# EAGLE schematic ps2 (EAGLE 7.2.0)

## Sheet 1 of 3: KL25Z Connections
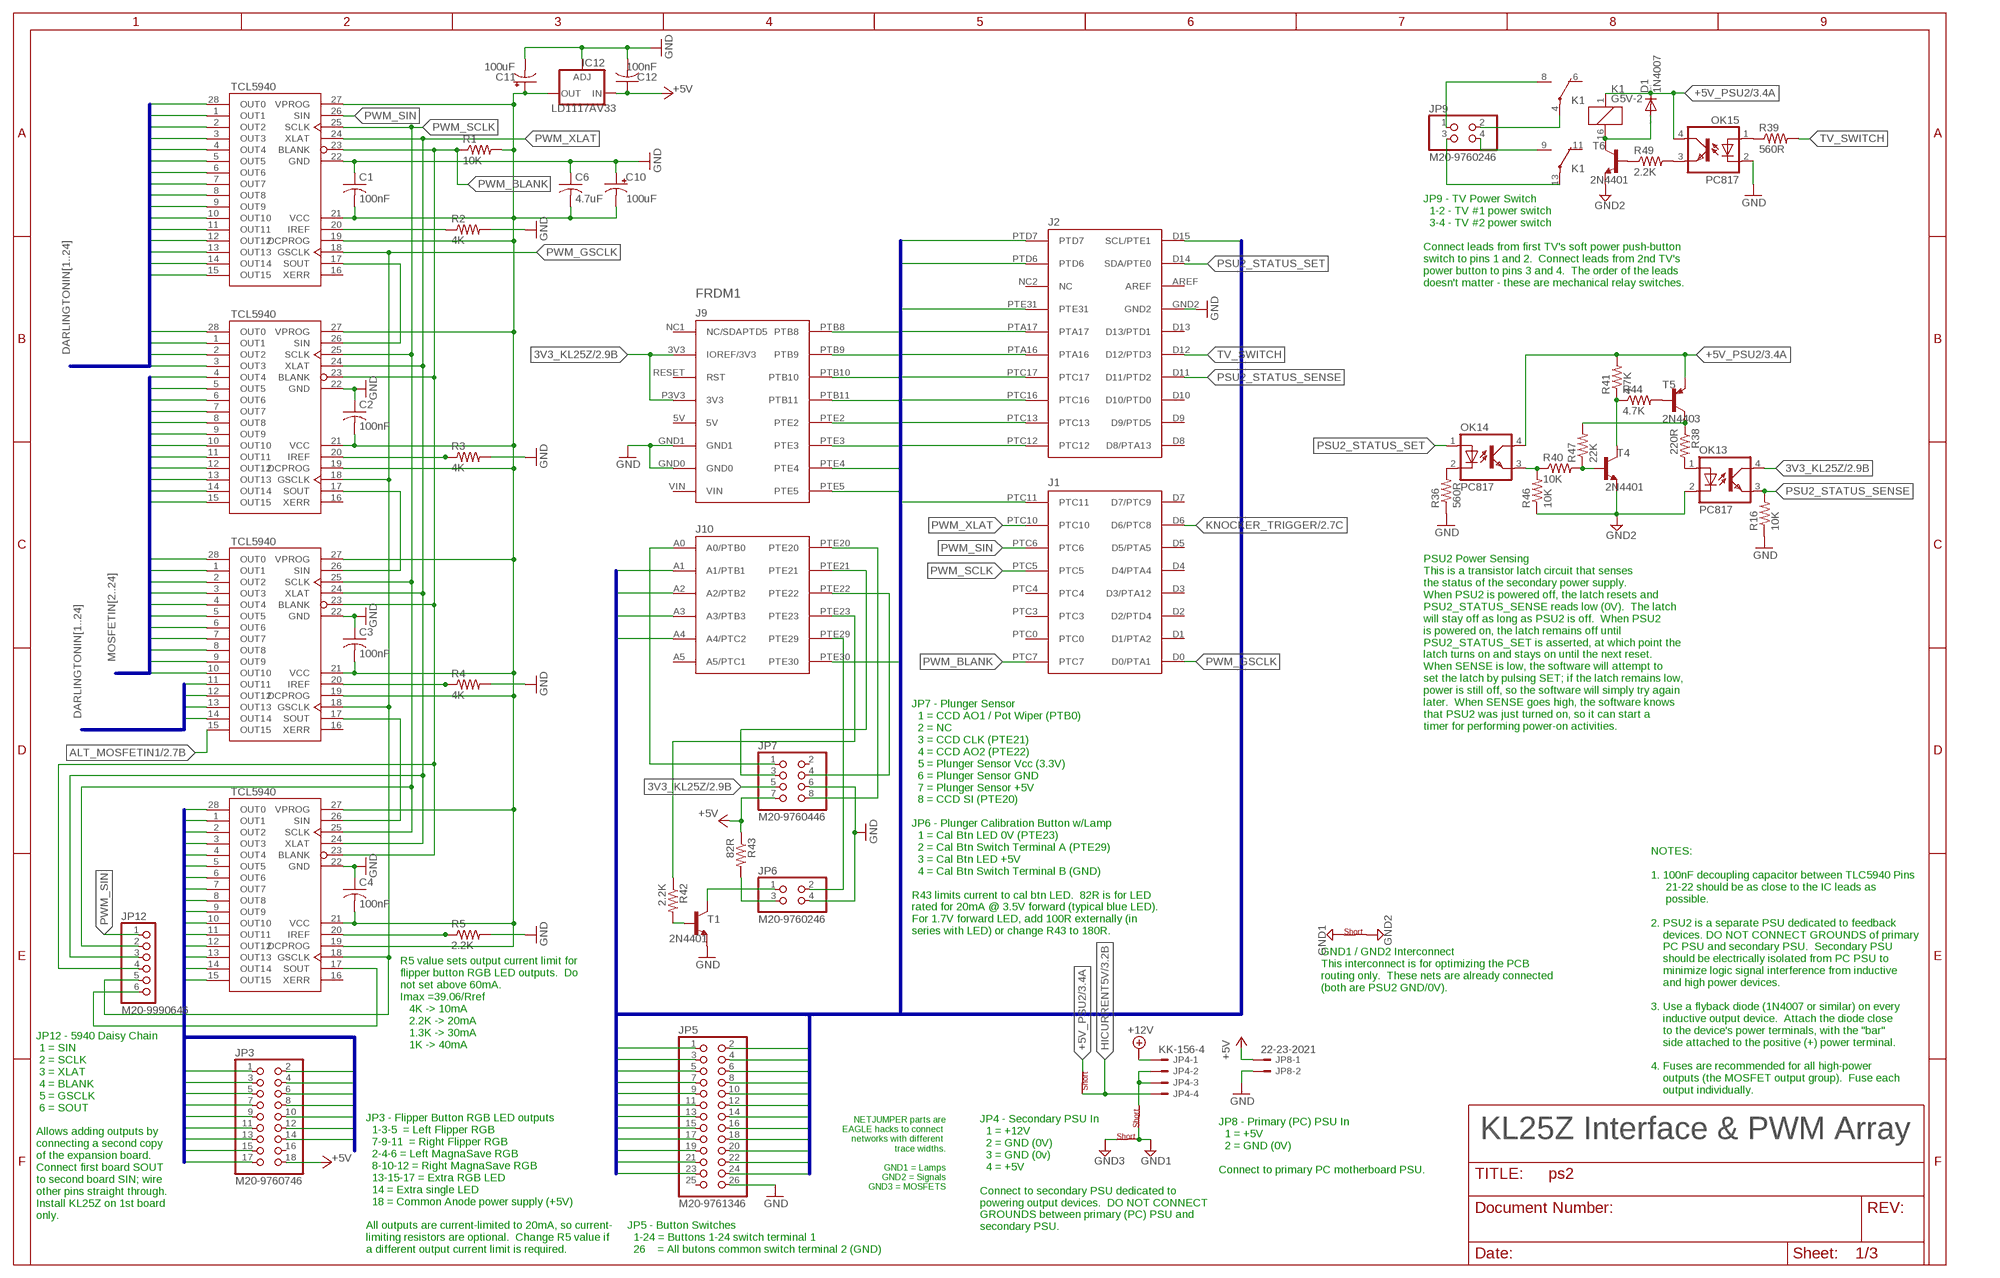
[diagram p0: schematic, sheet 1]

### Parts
C1  100nF  C-US025-024X044  [C025-024X044]
C2  100nF  C-US025-024X044  [C025-024X044]
C3  100nF  C-US025-024X044  [C025-024X044]
C4  100nF  C-US025-024X044  [C025-024X044]
C6  4.7uF  C-US025-024X044  [C025-024X044]
C10  100uF  CPOL-USE2.5-5  [E2,5-5]
C11  100uF  CPOL-USE2.5-5  [E2,5-5]
C12  100nF  C-US025-024X044  [C025-024X044]
D1  1N4007  DIODE-DO41-10  [DO41-10]
FRDM1  KL25Z  FRDM-KL25ZNORMAL  [FRDM_KL25Z_NORMAL]
IC1  TLC5940NT  TCL5940TLC5940NT  [DIP28]
IC2  TLC5940NT  TCL5940TLC5940NT  [DIP28]
IC3  TLC5940NT  TCL5940TLC5940NT  [DIP28]
IC4  TLC5940NT  TCL5940TLC5940NT  [DIP28]
IC12  LD1117AV33  LD117A  [TO220S]
JP3  M20-9760746  PINHD-2X9  [2X09]
JP4  KK-156-4  [KK-156-4]
JP5  M20-9761346  PINHD-2X13  [2X13]
JP6  M20-9760246  PINHD-2X2  [2X02]
JP7  M20-9760446  PINHD-2X4  [2X04]
JP8  22-23-2021  [22-23-2021]
JP9  M20-9760246  PINHD-2X2  [2X02]
JP12  M20-9990646  PINHD-1X6  [1X06]
K1  G5V-2  [G5V-2]
OK13  PC817  [DIL04]
OK14  PC817  [DIL04]
OK15  PC817  [DIL04]
R1  10K  R-US_0207/10  [0207/10]
R2  4K  R-US_0207/10  [0207/10]
R3  4K  R-US_0207/10  [0207/10]
R4  4K  R-US_0207/10  [0207/10]
R5  2.2K  R-US_0207/10  [0207/10]
R16  10K  R-US_0207/10  [0207/10]
R36  560R  R-US_0207/10  [0207/10]
R38  220R  R-US_0207/10  [0207/10]
R39  560R  R-US_0207/10  [0207/10]
R40  10K  R-US_0207/10  [0207/10]
R41  4.7K  R-US_0207/10  [0207/10]
R42  2.2K  R-US_0207/10  [0207/10]
R43  82R  R-US_0207/10  [0207/10]
R44  4.7K  R-US_0207/10  [0207/10]
R46  10K  R-US_0207/10  [0207/10]
R47  22K  R-US_0207/10  [0207/10]
R49  2.2K  R-US_0207/10  [0207/10]
T1  2N4401  2N4401-NPN-TO92-EBC  [TO92-EBC]
T4  2N4401  2N4401-NPN-TO92-EBC  [TO92-EBC]
T5  2N4403  2N4403-PNP-TO92-EBC  [TO92-EBC]
T6  2N4401  2N4401-NPN-TO92-EBC  [TO92-EBC]
U$1  NETJUMPER  [JP0]
U$2  NETJUMPER  [JP0]
U$3  NETJUMPER  [JP0]
U$4  NETJUMPER  [JP0]

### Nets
3V3_KL25Z: FRDM1.3V3(IOREF/3V3) FRDM1.P3V3(3V3) JP7.5 OK13.4(COL) ; also sheet 2
+5V [+5V]: C12.1 IC12.3(IN) JP3.18 JP7.7 JP8.1 R43.1 ; also sheet 2,3
+5V_PSU2: D1.C K1.1 OK14.4(COL) OK15.4(COL) R41.2 T5.E U$1.P$2 ; also sheet 3
+12V: JP4.1 ; also sheet 2
ALT_MOSFETIN1: IC3.15(OUT15) ; also sheet 2
DARLINGTONIN1: IC1.28(OUT0) ; also sheet 3
DARLINGTONIN2: IC1.1(OUT1) ; also sheet 3
DARLINGTONIN3: IC1.2(OUT2) ; also sheet 3
DARLINGTONIN4: IC1.3(OUT3) ; also sheet 3
DARLINGTONIN5: IC1.4(OUT4) ; also sheet 3
DARLINGTONIN6: IC1.5(OUT5) ; also sheet 3
DARLINGTONIN7: IC1.6(OUT6) ; also sheet 3
DARLINGTONIN8: IC1.7(OUT7) ; also sheet 3
DARLINGTONIN9: IC1.8(OUT8) ; also sheet 3
DARLINGTONIN10: IC1.9(OUT9) ; also sheet 3
DARLINGTONIN11: IC1.10(OUT10) ; also sheet 3
DARLINGTONIN12: IC1.11(OUT11) ; also sheet 3
DARLINGTONIN13: IC1.12(OUT12) ; also sheet 3
DARLINGTONIN14: IC1.13(OUT13) ; also sheet 3
DARLINGTONIN15: IC1.14(OUT14) ; also sheet 3
DARLINGTONIN16: IC1.15(OUT15) ; also sheet 3
DARLINGTONIN17: IC2.28(OUT0) ; also sheet 3
DARLINGTONIN18: IC2.1(OUT1) ; also sheet 3
DARLINGTONIN19: IC2.2(OUT2) ; also sheet 3
DARLINGTONIN20: IC2.3(OUT3) ; also sheet 3
DARLINGTONIN21: IC3.11(OUT11) ; also sheet 3
DARLINGTONIN22: IC3.12(OUT12) ; also sheet 3
DARLINGTONIN23: IC3.13(OUT13) ; also sheet 3
DARLINGTONIN24: IC3.14(OUT14) ; also sheet 3
FLIPPER_RGB1: IC4.28(OUT0) JP3.1
FLIPPER_RGB2: IC4.1(OUT1) JP3.3
FLIPPER_RGB3: IC4.2(OUT2) JP3.5
FLIPPER_RGB4: IC4.3(OUT3) JP3.7
FLIPPER_RGB5: IC4.4(OUT4) JP3.9
FLIPPER_RGB6: IC4.5(OUT5) JP3.11
FLIPPER_RGB7: IC4.6(OUT6) JP3.2
FLIPPER_RGB8: IC4.7(OUT7) JP3.4
FLIPPER_RGB9: IC4.8(OUT8) JP3.6
FLIPPER_RGB10: IC4.9(OUT9) JP3.8
FLIPPER_RGB11: IC4.10(OUT10) JP3.10
FLIPPER_RGB12: IC4.11(OUT11) JP3.12
FLIPPER_RGB13: IC4.12(OUT12) JP3.13
FLIPPER_RGB14: IC4.13(OUT13) JP3.15
FLIPPER_RGB15: IC4.14(OUT14) JP3.17
FLIPPER_RGB16: IC4.15(OUT15) JP3.14
GND [GND]: C1.1 C2.1 C3.1 C4.1 C6.1 C10.+ C11.- C12.2 FRDM1.GND0 FRDM1.GND1 FRDM1.GND2 IC1.22(GND) IC2.22(GND) IC3.22(GND) IC4.22(GND) IC12.1(ADJ) JP5.26 JP6.4 JP7.6 JP8.2 OK15.2(C) R2.2 R3.2 R4.2 R5.2 R16.1 R36.1 T1.E ; also sheet 2
GND1 [Lamp Power & Ground]: U$2.P$2 U$3.P$2 U$4.P$1 ; also sheet 3
GND2: OK13.2(C) R46.1 T4.E T6.E U$3.P$1
GND3 [MOSFET Power & Ground]: U$4.P$2 ; also sheet 2
HICURRENT5V [Lamp Power & Ground]: JP4.4 U$1.P$1 ; also sheet 3
KEYS1: FRDM1.A4(A4/PTC2) JP5.1
KEYS2: FRDM1.A3(A3/PTB3) JP5.2
KEYS3: FRDM1.A2(A2/PTB2) JP5.3
KEYS4: FRDM1.A1(A1/PTB1) JP5.4
KEYS5: FRDM1.PTE30 JP5.5
KEYS6: FRDM1.PTC11 JP5.6
KEYS7: FRDM1.PTE5 JP5.7
KEYS8: FRDM1.PTE4 JP5.8
KEYS9: FRDM1.PTE3 JP5.9
KEYS10: FRDM1.PTE2 JP5.10
KEYS11: FRDM1.PTB11 JP5.11
KEYS12: FRDM1.PTB10 JP5.12
KEYS13: FRDM1.PTB9 JP5.13
KEYS14: FRDM1.PTB8 JP5.14
KEYS15: FRDM1.PTC12 JP5.15
KEYS16: FRDM1.PTC13 JP5.16
KEYS17: FRDM1.PTC16 JP5.17
KEYS18: FRDM1.PTC17 JP5.18
KEYS19: FRDM1.PTA16 JP5.19
KEYS20: FRDM1.PTA17 JP5.20
KEYS21: FRDM1.PTE31 JP5.21
KEYS22: FRDM1.PTD6 JP5.22
KEYS23: FRDM1.PTD7 JP5.23
KEYS24: FRDM1.D15(SCL/PTE1) JP5.24
KNOCKER_TRIGGER: FRDM1.D6(D6/PTC8) ; also sheet 2
MOSFETIN2: IC2.4(OUT4) ; also sheet 2
MOSFETIN3: IC2.5(OUT5) ; also sheet 2
MOSFETIN4: IC2.6(OUT6) ; also sheet 2
MOSFETIN5: IC2.7(OUT7) ; also sheet 2
MOSFETIN6: IC2.8(OUT8) ; also sheet 2
MOSFETIN7: IC2.9(OUT9) ; also sheet 2
MOSFETIN8: IC2.10(OUT10) ; also sheet 2
MOSFETIN9: IC2.11(OUT11) ; also sheet 2
MOSFETIN10: IC2.12(OUT12) ; also sheet 2
MOSFETIN11: IC2.13(OUT13) ; also sheet 2
MOSFETIN12: IC2.14(OUT14) ; also sheet 2
MOSFETIN13: IC2.15(OUT15) ; also sheet 2
MOSFETIN14: IC3.28(OUT0) ; also sheet 2
MOSFETIN15: IC3.1(OUT1) ; also sheet 2
MOSFETIN16: IC3.2(OUT2) ; also sheet 2
MOSFETIN17: IC3.3(OUT3) ; also sheet 2
MOSFETIN18: IC3.4(OUT4) ; also sheet 2
MOSFETIN19: IC3.5(OUT5) ; also sheet 2
MOSFETIN20: IC3.6(OUT6) ; also sheet 2
MOSFETIN21: IC3.7(OUT7) ; also sheet 2
MOSFETIN22: IC3.8(OUT8) ; also sheet 2
MOSFETIN23: IC3.9(OUT9) ; also sheet 2
MOSFETIN24: IC3.10(OUT10) ; also sheet 2
N$1: IC1.17(SOUT) IC2.26(SIN)
N$2: IC2.17(SOUT) IC3.26(SIN)
N$3: IC3.17(SOUT) IC4.26(SIN)
N$5: OK15.1(A) R39.1
N$8: R38.1 R47.2 T5.C
N$10: OK13.1(A) R38.2
N$11: OK15.3(EMIT) R49.2
N$12: R49.1 T6.B
N$13: R44.2 T5.B
N$14: R41.1 R44.1 T4.C
N$15: D1.A K1.16 T6.C
N$16: JP9.2 K1.4(1:P)
N$17: IC1.20(IREF) R2.1
N$18: IC2.20(IREF) R3.1
N$19: IC3.20(IREF) R4.1
N$20: IC4.20(IREF) R5.1
N$21: FRDM1.A0(A0/PTB0) JP7.1
N$26: FRDM1.PTE20 JP7.8
N$34: FRDM1.PTE21 JP7.3
N$38: FRDM1.PTE29 JP6.2
N$41: FRDM1.PTE23 R42.1
N$43: OK14.3(EMIT) R40.1 R46.2
N$50: JP9.1 K1.8(1:S)
N$61: OK14.2(C) R36.2
N$68: C1.2 C2.2 C3.2 C4.2 C6.2 C10.- C11.+ IC1.19(DCPROG) IC1.21(VCC) IC1.27(VPROG) IC2.19(DCPROG) IC2.21(VCC) IC2.27(VPROG) IC3.19(DCPROG) IC3.21(VCC) IC3.27(VPROG) IC4.19(DCPROG) IC4.21(VCC) IC4.27(VPROG) IC12.2(OUT) R1.2
N$70: JP4.2 JP4.3 U$2.P$1
N$75: FRDM1.PTE22 JP7.4
N$76: IC4.17(SOUT) JP12.6
N$85: R40.2 R47.1 T4.B
N$86: JP9.4 K1.9(2:S)
N$87: JP9.3 K1.13(2:P)
N$88 [+5V]: JP6.3 R43.2
N$89: JP6.1 T1.C
N$100: R42.2 T1.B
PSU2_STATUS_SENSE: FRDM1.D11(D11/PTD2) OK13.3(EMIT) R16.2
PSU2_STATUS_SET: FRDM1.D14(SDA/PTE0) OK14.1(A)
PWM_BLANK: FRDM1.PTC7 IC1.23(BLANK) IC2.23(BLANK) IC3.23(BLANK) IC4.23(BLANK) JP12.4 R1.1
PWM_GSCLK: FRDM1.D0(D0/PTA1) IC1.18(GSCLK) IC2.18(GSCLK) IC3.18(GSCLK) IC4.18(GSCLK) JP12.5
PWM_SCLK: FRDM1.PTC5 IC1.25(SCLK) IC2.25(SCLK) IC3.25(SCLK) IC4.25(SCLK) JP12.2
PWM_SIN: FRDM1.PTC6 IC1.26(SIN) JP12.1
PWM_XLAT: FRDM1.PTC10 IC1.24(XLAT) IC2.24(XLAT) IC3.24(XLAT) IC4.24(XLAT) JP12.3
TV_SWITCH: FRDM1.D12(D12/PTD3) R39.2
Unconnected: FRDM1.5V FRDM1.A5(A5/PTC1) FRDM1.AREF FRDM1.D1(D1/PTA2) FRDM1.D2(D2/PTD4) FRDM1.D3(D3/PTA12) FRDM1.D4(D4/PTA4) FRDM1.D5(D5/PTA5) FRDM1.D7(D7/PTC9) FRDM1.D8(D8/PTA13) FRDM1.D9(D9/PTD5) FRDM1.D10(D10/PTD0) FRDM1.D13(D13/PTD1) FRDM1.NC1(NC/SDAPTD5) FRDM1.NC2(NC) FRDM1.PTC0 FRDM1.PTC3 FRDM1.PTC4 FRDM1.RESET(RST) FRDM1.VIN IC1.16(XERR) IC2.16(XERR) IC3.16(XERR) IC4.16(XERR) JP3.16 JP5.25 JP7.2 K1.6(1:O) K1.11(2:O)

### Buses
FLIPPER_RGB[1..17]
KEYS[1..24]
MOSFETIN[2..24]
DARLINGTONIN[1..24]

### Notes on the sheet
- JP9 - TV Power Switch
    1-2 - TV #1 power switch
    3-4 - TV #2 power switch
  
  Connect leads from first TV's soft power push-button
  switch to pins 1 and 2.  Connect leads from 2nd TV's
  power button to pins 3 and 4.  The order of the leads
  doesn't matter - these are mechanical relay switches.
- PSU2 Power Sensing
  This is a transistor latch circuit that senses
  the status of the secondary power supply.
  When PSU2 is powered off, the latch resets and
  PSU2_STATUS_SENSE reads low (0V).  The latch
  will stay off as long as PSU2 is off.  When PSU2
  is powered on, the latch remains off until 
  PSU2_STATUS_SET is asserted, at which point the
  latch turns on and stays on until the next reset.
  When SENSE is low, the software will attempt to
  set the latch by pulsing SET; if the latch remains low,
  power is still off, so the software will simply try again
  later.  When SENSE goes high, the software knows
  that PSU2 was just turned on, so it can start a
  timer for performing power-on activities.
- JP7 - Plunger Sensor
    1 = CCD AO1 / Pot Wiper (PTB0)
    2 = NC
    3 = CCD CLK (PTE21)
    4 = CCD AO2 (PTE22)
    5 = Plunger Sensor Vcc (3.3V)
    6 = Plunger Sensor GND
    7 = Plunger Sensor +5V
    8 = CCD SI (PTE20)
  
  JP6 - Plunger Calibration Button w/Lamp
    1 = Cal Btn LED 0V (PTE23)
    2 = Cal Btn Switch Terminal A (PTE29)
    3 = Cal Btn LED +5V
    4 = Cal Btn Switch Terminal B (GND)
  
  R43 limits current to cal btn LED.  82R is for LED
  rated for 20mA @ 3.5V forward (typical blue LED).
  For 1.7V forward LED, add 100R externally (in
  series with LED) or change R43 to 180R.
- GND1 / GND2 Interconnect
  This interconnect is for optimizing the PCB 
  routing only.  These nets are already connected
  (both are PSU2 GND/0V).
- R5 value sets output current limit for 
  flipper button RGB LED outputs.  Do
  not set above 60mA.
  Imax =39.06/Rref
     4K -> 10mA
     2.2K -> 20mA
     1.3K -> 30mA
     1K -> 40mA
- NOTES:
  
  1. 100nF decoupling capacitor between TLC5940 Pins
       21-22 should be as close to the IC leads as 
       possible.
  
  2. PSU2 is a separate PSU dedicated to feedback
      devices. DO NOT CONNECT GROUNDS of primary
      PC PSU and secondary PSU.  Secondary PSU 
      should be electrically isolated from PC PSU to
      minimize logic signal interference from inductive 
      and high power devices.
  
  3. Use a flyback diode (1N4007 or similar) on every
      inductive output device.  Attach the diode close
      to the device's power terminals, with the "bar"
      side attached to the positive (+) power terminal.
  
  4. Fuses are recommended for all high-power
      outputs (the MOSFET output group).  Fuse each
      output individually.
- NETJUMPER parts are
  EAGLE hacks to connect 
  networks with different 
  trace widths.
  
  GND1 = Lamps
  GND2 = Signals
  GND3 = MOSFETS
- KL25Z Interface & PWM Array
- JP8 - Primary (PC) PSU In
    1 = +5V
    2 = GND (0V)
  
  Connect to primary PC motherboard PSU.
- JP12 - 5940 Daisy Chain
   1 = SIN
   2 = SCLK
   3 = XLAT
   4 = BLANK
   5 = GSCLK
   6 = SOUT
  
  Allows adding outputs by
  connecting a second copy
  of the expansion board.
  Connect first board SOUT
  to second board SIN; wire
  other pins straight through.
  Install KL25Z on 1st board
  only.
- JP4 - Secondary PSU In
    1 = +12V
    2 = GND (0V)
    3 = GND (0v)
    4 = +5V
  
  Connect to secondary PSU dedicated to
  powering output devices.  DO NOT CONNECT
  GROUNDS between primary (PC) PSU and
  secondary PSU.
- JP3 - Flipper Button RGB LED outputs
    1-3-5  = Left Flipper RGB
    7-9-11  = Right Flipper RGB
    2-4-6 = Left MagnaSave RGB
    8-10-12 = Right MagnaSave RGB
    13-15-17 = Extra RGB LED
    14 = Extra single LED
    18 = Common Anode power supply (+5V)
  
  All outputs are current-limited to 20mA, so current-
  limiting resistors are optional.  Change R5 value if
  a different output current limit is required.
- JP5 - Button Switches
    1-24 = Buttons 1-24 switch terminal 1
    26    = All butons common switch terminal 2 (GND)

## Sheet 2 of 3: MOSFET Outputs
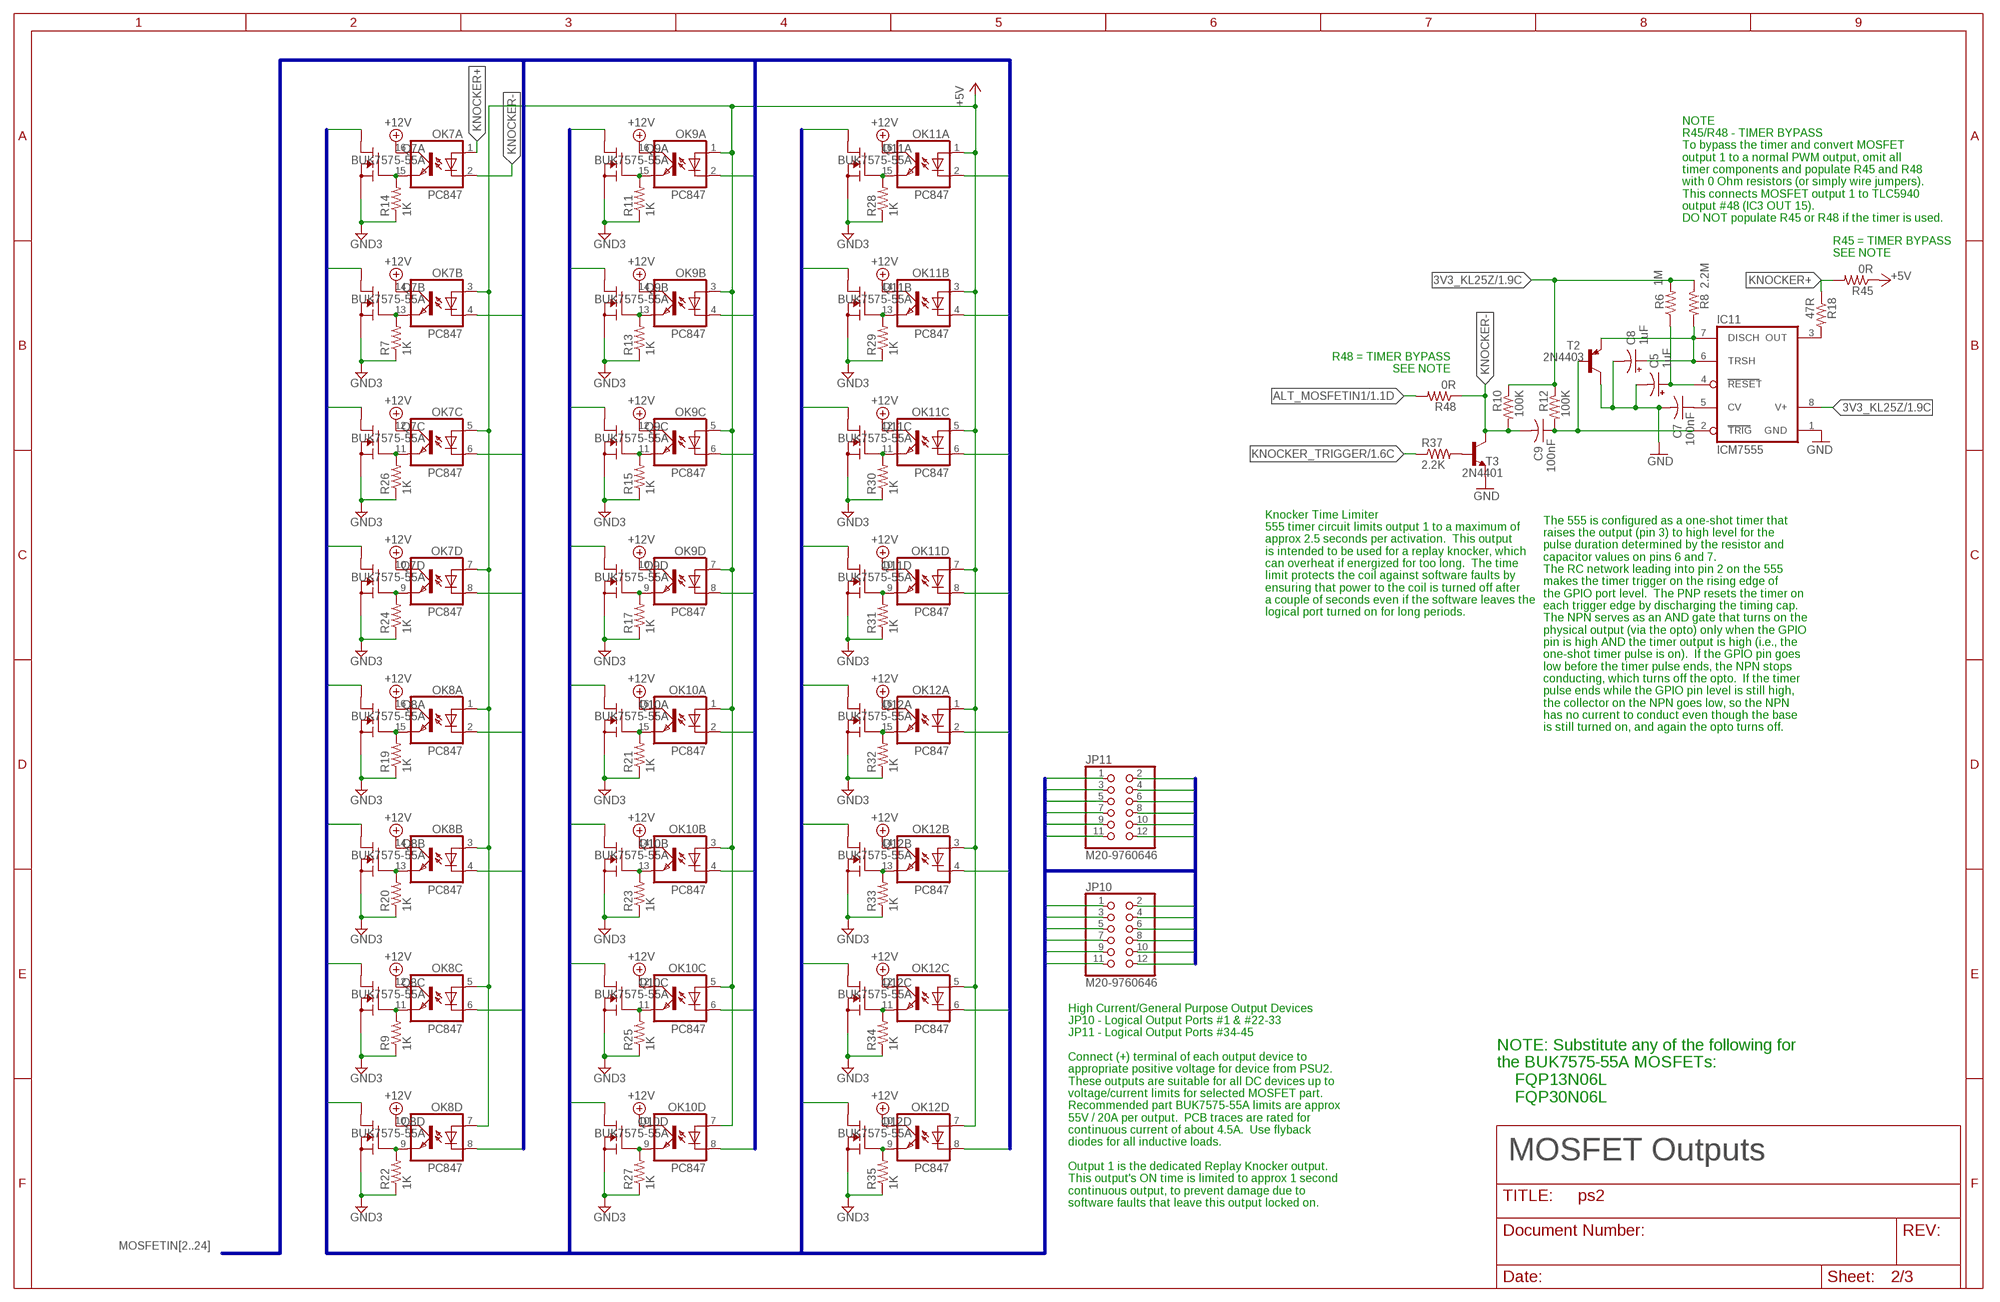
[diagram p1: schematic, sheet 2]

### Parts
C5  1uF  CPOL-USE2.5-5  [E2,5-5]
C7  100nF  C-US025-024X044  [C025-024X044]
C8  1uF  CPOL-USE2.5-5  [E2,5-5]
C9  100nF  C-US025-024X044  [C025-024X044]
IC11  ICM7555  [DIL08]
JP10  M20-9760646  PINHD-2X6  [2X06]
JP11  M20-9760646  PINHD-2X6  [2X06]
OK7  PC847  [DIL16]
OK8  PC847  [DIL16]
OK9  PC847  [DIL16]
OK10  PC847  [DIL16]
OK11  PC847  [DIL16]
OK12  PC847  [DIL16]
Q7A  BUK7575-55A  [TO220BV]
Q7B  BUK7575-55A  [TO220BV]
Q7C  BUK7575-55A  [TO220BV]
Q7D  BUK7575-55A  [TO220BV]
Q8A  BUK7575-55A  [TO220BV]
Q8B  BUK7575-55A  [TO220BV]
Q8C  BUK7575-55A  [TO220BV]
Q8D  BUK7575-55A  [TO220BV]
Q9A  BUK7575-55A  [TO220BV]
Q9B  BUK7575-55A  [TO220BV]
Q9C  BUK7575-55A  [TO220BV]
Q9D  BUK7575-55A  [TO220BV]
Q10A  BUK7575-55A  [TO220BV]
Q10B  BUK7575-55A  [TO220BV]
Q10C  BUK7575-55A  [TO220BV]
Q10D  BUK7575-55A  [TO220BV]
Q11A  BUK7575-55A  [TO220BV]
Q11B  BUK7575-55A  [TO220BV]
Q11C  BUK7575-55A  [TO220BV]
Q11D  BUK7575-55A  [TO220BV]
Q12A  BUK7575-55A  [TO220BV]
Q12B  BUK7575-55A  [TO220BV]
Q12C  BUK7575-55A  [TO220BV]
Q12D  BUK7575-55A  [TO220BV]
R6  1M  R-US_0207/10  [0207/10]
R7  1K  R-US_0207/10  [0207/10]
R8  2.2M  R-US_0207/10  [0207/10]
R9  1K  R-US_0207/10  [0207/10]
R10  100K  R-US_0207/10  [0207/10]
R11  1K  R-US_0207/10  [0207/10]
R12  100K  R-US_0207/10  [0207/10]
R13  1K  R-US_0207/10  [0207/10]
R14  1K  R-US_0207/10  [0207/10]
R15  1K  R-US_0207/10  [0207/10]
R17  1K  R-US_0207/10  [0207/10]
R18  47R  R-US_0207/10  [0207/10]
R19  1K  R-US_0207/10  [0207/10]
R20  1K  R-US_0207/10  [0207/10]
R21  1K  R-US_0207/10  [0207/10]
R22  1K  R-US_0207/10  [0207/10]
R23  1K  R-US_0207/10  [0207/10]
R24  1K  R-US_0207/10  [0207/10]
R25  1K  R-US_0207/10  [0207/10]
R26  1K  R-US_0207/10  [0207/10]
R27  1K  R-US_0207/10  [0207/10]
R28  1K  R-US_0207/10  [0207/10]
R29  1K  R-US_0207/10  [0207/10]
R30  1K  R-US_0207/10  [0207/10]
R31  1K  R-US_0207/10  [0207/10]
R32  1K  R-US_0207/10  [0207/10]
R33  1K  R-US_0207/10  [0207/10]
R34  1K  R-US_0207/10  [0207/10]
R35  1K  R-US_0207/10  [0207/10]
R37  2.2K  R-US_0207/10  [0207/10]
R45  0R  R-US_0204/2V  [0204V]
R48  0R  R-US_0204/2V  [0204V]
T2  2N4403  2N4403-PNP-TO92-EBC  [TO92-EBC]
T3  2N4401  2N4401-NPN-TO92-EBC  [TO92-EBC]

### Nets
3V3_KL25Z: IC11.8(V+) R6.2 R8.1 R10.1 R12.1 ; also sheet 1
+5V [+5V]: OK7.3(B:A) OK7.5(C:A) OK7.7(D:A) OK8.1(A:A) OK8.3(B:A) OK8.5(C:A) OK8.7(D:A) OK9.1(A:A) OK9.3(B:A) OK9.5(C:A) OK9.7(D:A) OK10.1(A:A) OK10.3(B:A) OK10.5(C:A) OK10.7(D:A) OK11.1(A:A) OK11.3(B:A) OK11.5(C:A) OK11.7(D:A) OK12.1(A:A) OK12.3(B:A) OK12.5(C:A) OK12.7(D:A) R45.1 ; also sheet 1,3
+12V: OK7.10(D:COL) OK7.12(C:COL) OK7.14(B:COL) OK7.16(A:COL) OK8.10(D:COL) OK8.12(C:COL) OK8.14(B:COL) OK8.16(A:COL) OK9.10(D:COL) OK9.12(C:COL) OK9.14(B:COL) OK9.16(A:COL) OK10.10(D:COL) OK10.12(C:COL) OK10.14(B:COL) OK10.16(A:COL) OK11.10(D:COL) OK11.12(C:COL) OK11.14(B:COL) OK11.16(A:COL) OK12.10(D:COL) OK12.12(C:COL) OK12.14(B:COL) OK12.16(A:COL) ; also sheet 1
ALT_MOSFETIN1: R48.2 ; also sheet 1
GND [GND]: C5.- C7.2 C8.- IC11.1(GND) T2.C T3.E ; also sheet 1
GND3 [MOSFET Power & Ground]: Q7A.3(S) Q7B.3(S) Q7C.3(S) Q7D.3(S) Q8A.3(S) Q8B.3(S) Q8C.3(S) Q8D.3(S) Q9A.3(S) Q9B.3(S) Q9C.3(S) Q9D.3(S) Q10A.3(S) Q10B.3(S) Q10C.3(S) Q10D.3(S) Q11A.3(S) Q11B.3(S) Q11C.3(S) Q11D.3(S) Q12A.3(S) Q12B.3(S) Q12C.3(S) Q12D.3(S) R7.1 R9.1 R11.1 R13.1 R14.1 R15.1 R17.1 R19.1 R20.1 R21.1 R22.1 R23.1 R24.1 R25.1 R26.1 R27.1 R28.1 R29.1 R30.1 R31.1 R32.1 R33.1 R34.1 R35.1 ; also sheet 1
KNOCKER+: OK7.1(A:A) R18.1 R45.2
KNOCKER-: C9.2 OK7.2(A:C) R10.2 R48.1 T3.C
KNOCKER_TRIGGER: R37.1 ; also sheet 1
MOSFETIN2: OK7.4(B:C) ; also sheet 1
MOSFETIN3: OK7.6(C:C) ; also sheet 1
MOSFETIN4: OK7.8(D:C) ; also sheet 1
MOSFETIN5: OK8.2(A:C) ; also sheet 1
MOSFETIN6: OK8.4(B:C) ; also sheet 1
MOSFETIN7: OK8.6(C:C) ; also sheet 1
MOSFETIN8: OK8.8(D:C) ; also sheet 1
MOSFETIN9: OK9.2(A:C) ; also sheet 1
MOSFETIN10: OK9.4(B:C) ; also sheet 1
MOSFETIN11: OK9.6(C:C) ; also sheet 1
MOSFETIN12: OK9.8(D:C) ; also sheet 1
MOSFETIN13: OK10.2(A:C) ; also sheet 1
MOSFETIN14: OK10.4(B:C) ; also sheet 1
MOSFETIN15: OK10.6(C:C) ; also sheet 1
MOSFETIN16: OK10.8(D:C) ; also sheet 1
MOSFETIN17: OK11.2(A:C) ; also sheet 1
MOSFETIN18: OK11.4(B:C) ; also sheet 1
MOSFETIN19: OK11.6(C:C) ; also sheet 1
MOSFETIN20: OK11.8(D:C) ; also sheet 1
MOSFETIN21: OK12.2(A:C) ; also sheet 1
MOSFETIN22: OK12.4(B:C) ; also sheet 1
MOSFETIN23: OK12.6(C:C) ; also sheet 1
MOSFETIN24: OK12.8(D:C) ; also sheet 1
MOSFETOUT1 [MOSFET Power & Ground]: JP10.1 Q7A.2(D)
MOSFETOUT2 [MOSFET Power & Ground]: JP10.2 Q7B.2(D)
MOSFETOUT3 [MOSFET Power & Ground]: JP10.3 Q7C.2(D)
MOSFETOUT4 [MOSFET Power & Ground]: JP10.4 Q7D.2(D)
MOSFETOUT5 [MOSFET Power & Ground]: JP10.5 Q8A.2(D)
MOSFETOUT6 [MOSFET Power & Ground]: JP10.6 Q8B.2(D)
MOSFETOUT7 [MOSFET Power & Ground]: JP10.7 Q8C.2(D)
MOSFETOUT8 [MOSFET Power & Ground]: JP10.8 Q8D.2(D)
MOSFETOUT9 [MOSFET Power & Ground]: JP10.9 Q9A.2(D)
MOSFETOUT10 [MOSFET Power & Ground]: JP10.10 Q9B.2(D)
MOSFETOUT11 [MOSFET Power & Ground]: JP10.11 Q9C.2(D)
MOSFETOUT12 [MOSFET Power & Ground]: JP10.12 Q9D.2(D)
MOSFETOUT13 [MOSFET Power & Ground]: JP11.1 Q10A.2(D)
MOSFETOUT14 [MOSFET Power & Ground]: JP11.2 Q10B.2(D)
MOSFETOUT15 [MOSFET Power & Ground]: JP11.3 Q10C.2(D)
MOSFETOUT16 [MOSFET Power & Ground]: JP11.4 Q10D.2(D)
MOSFETOUT17 [MOSFET Power & Ground]: JP11.5 Q11A.2(D)
MOSFETOUT18 [MOSFET Power & Ground]: JP11.6 Q11B.2(D)
MOSFETOUT19 [MOSFET Power & Ground]: JP11.7 Q11C.2(D)
MOSFETOUT20 [MOSFET Power & Ground]: JP11.8 Q11D.2(D)
MOSFETOUT21 [MOSFET Power & Ground]: JP11.9 Q12A.2(D)
MOSFETOUT22 [MOSFET Power & Ground]: JP11.10 Q12B.2(D)
MOSFETOUT23 [MOSFET Power & Ground]: JP11.11 Q12C.2(D)
MOSFETOUT24 [MOSFET Power & Ground]: JP11.12 Q12D.2(D)
N$4: IC11.3(OUT) R18.2
N$6: C5.+ IC11.4(RESET) R6.1
N$9: R37.2 T3.B
N$42: OK7.13(B:EMIT) Q7B.1(G) R7.2
N$44: OK8.11(C:EMIT) Q8C.1(G) R9.2
N$45: OK8.9(D:EMIT) Q8D.1(G) R22.2
N$46: OK8.15(A:EMIT) Q8A.1(G) R19.2
N$47: OK8.13(B:EMIT) Q8B.1(G) R20.2
N$48: OK7.9(D:EMIT) Q7D.1(G) R24.2
N$49: OK7.11(C:EMIT) Q7C.1(G) R26.2
N$51: OK9.15(A:EMIT) Q9A.1(G) R11.2
N$52: OK9.13(B:EMIT) Q9B.1(G) R13.2
N$53: OK9.11(C:EMIT) Q9C.1(G) R15.2
N$54: OK9.9(D:EMIT) Q9D.1(G) R17.2
N$55: OK10.15(A:EMIT) Q10A.1(G) R21.2
N$56: OK10.13(B:EMIT) Q10B.1(G) R23.2
N$57: OK10.11(C:EMIT) Q10C.1(G) R25.2
N$58: OK10.9(D:EMIT) Q10D.1(G) R27.2
N$59: OK11.15(A:EMIT) Q11A.1(G) R28.2
N$60: OK11.13(B:EMIT) Q11B.1(G) R29.2
N$62: OK11.11(C:EMIT) Q11C.1(G) R30.2
N$63: OK11.9(D:EMIT) Q11D.1(G) R31.2
N$64: OK12.15(A:EMIT) Q12A.1(G) R32.2
N$65: OK12.13(B:EMIT) Q12B.1(G) R33.2
N$66: OK12.11(C:EMIT) Q12C.1(G) R34.2
N$67: OK12.9(D:EMIT) Q12D.1(G) R35.2
N$69: C7.1 IC11.5(CV)
N$71: C8.+ IC11.6(TRSH) IC11.7(DISCH) R8.2 T2.E
N$72: OK7.15(A:EMIT) Q7A.1(G) R14.2
N$74: C9.1 IC11.2(TRIG) R12.2 T2.B

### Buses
MOSFETIN[2..24]
MOSFETOUT[1..24]

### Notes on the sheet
- NOTE
  R45/R48 - TIMER BYPASS
  To bypass the timer and convert MOSFET
  output 1 to a normal PWM output, omit all
  timer components and populate R45 and R48
  with 0 Ohm resistors (or simply wire jumpers).
  This connects MOSFET output 1 to TLC5940
  output #48 (IC3 OUT 15).
  DO NOT populate R45 or R48 if the timer is used.
- R45 = TIMER BYPASS
  SEE NOTE
- R48 = TIMER BYPASS
  SEE NOTE
- Knocker Time Limiter
  555 timer circuit limits output 1 to a maximum of
  approx 2.5 seconds per activation.  This output
  is intended to be used for a replay knocker, which
  can overheat if energized for too long.  The time
  limit protects the coil against software faults by
  ensuring that power to the coil is turned off after
  a couple of seconds even if the software leaves the
  logical port turned on for long periods.
- The 555 is configured as a one-shot timer that
  raises the output (pin 3) to high level for the
  pulse duration determined by the resistor and
  capacitor values on pins 6 and 7.
  The RC network leading into pin 2 on the 555
  makes the timer trigger on the rising edge of
  the GPIO port level.  The PNP resets the timer on
  each trigger edge by discharging the timing cap. 
  The NPN serves as an AND gate that turns on the
  physical output (via the opto) only when the GPIO
  pin is high AND the timer output is high (i.e., the
  one-shot timer pulse is on).  If the GPIO pin goes
  low before the timer pulse ends, the NPN stops
  conducting, which turns off the opto.  If the timer
  pulse ends while the GPIO pin level is still high,
  the collector on the NPN goes low, so the NPN
  has no current to conduct even though the base
  is still turned on, and again the opto turns off.
- NOTE: Substitute any of the following for
  the BUK7575-55A MOSFETs:
      FQP13N06L
      FQP30N06L
- MOSFET Outputs
- High Current/General Purpose Output Devices
  JP10 - Logical Output Ports #1 & #22-33
  JP11 - Logical Output Ports #34-45
  
  Connect (+) terminal of each output device to
  appropriate positive voltage for device from PSU2.
  These outputs are suitable for all DC devices up to
  voltage/current limits for selected MOSFET part.
  Recommended part BUK7575-55A limits are approx
  55V / 20A per output.  PCB traces are rated for
  continuous current of about 4.5A.  Use flyback 
  diodes for all inductive loads.
  
  Output 1 is the dedicated Replay Knocker output.
  This output's ON time is limited to approx 1 second
  continuous output, to prevent damage due to
  software faults that leave this output locked on.

## Sheet 3 of 3: Flasher/Lamp Outputs
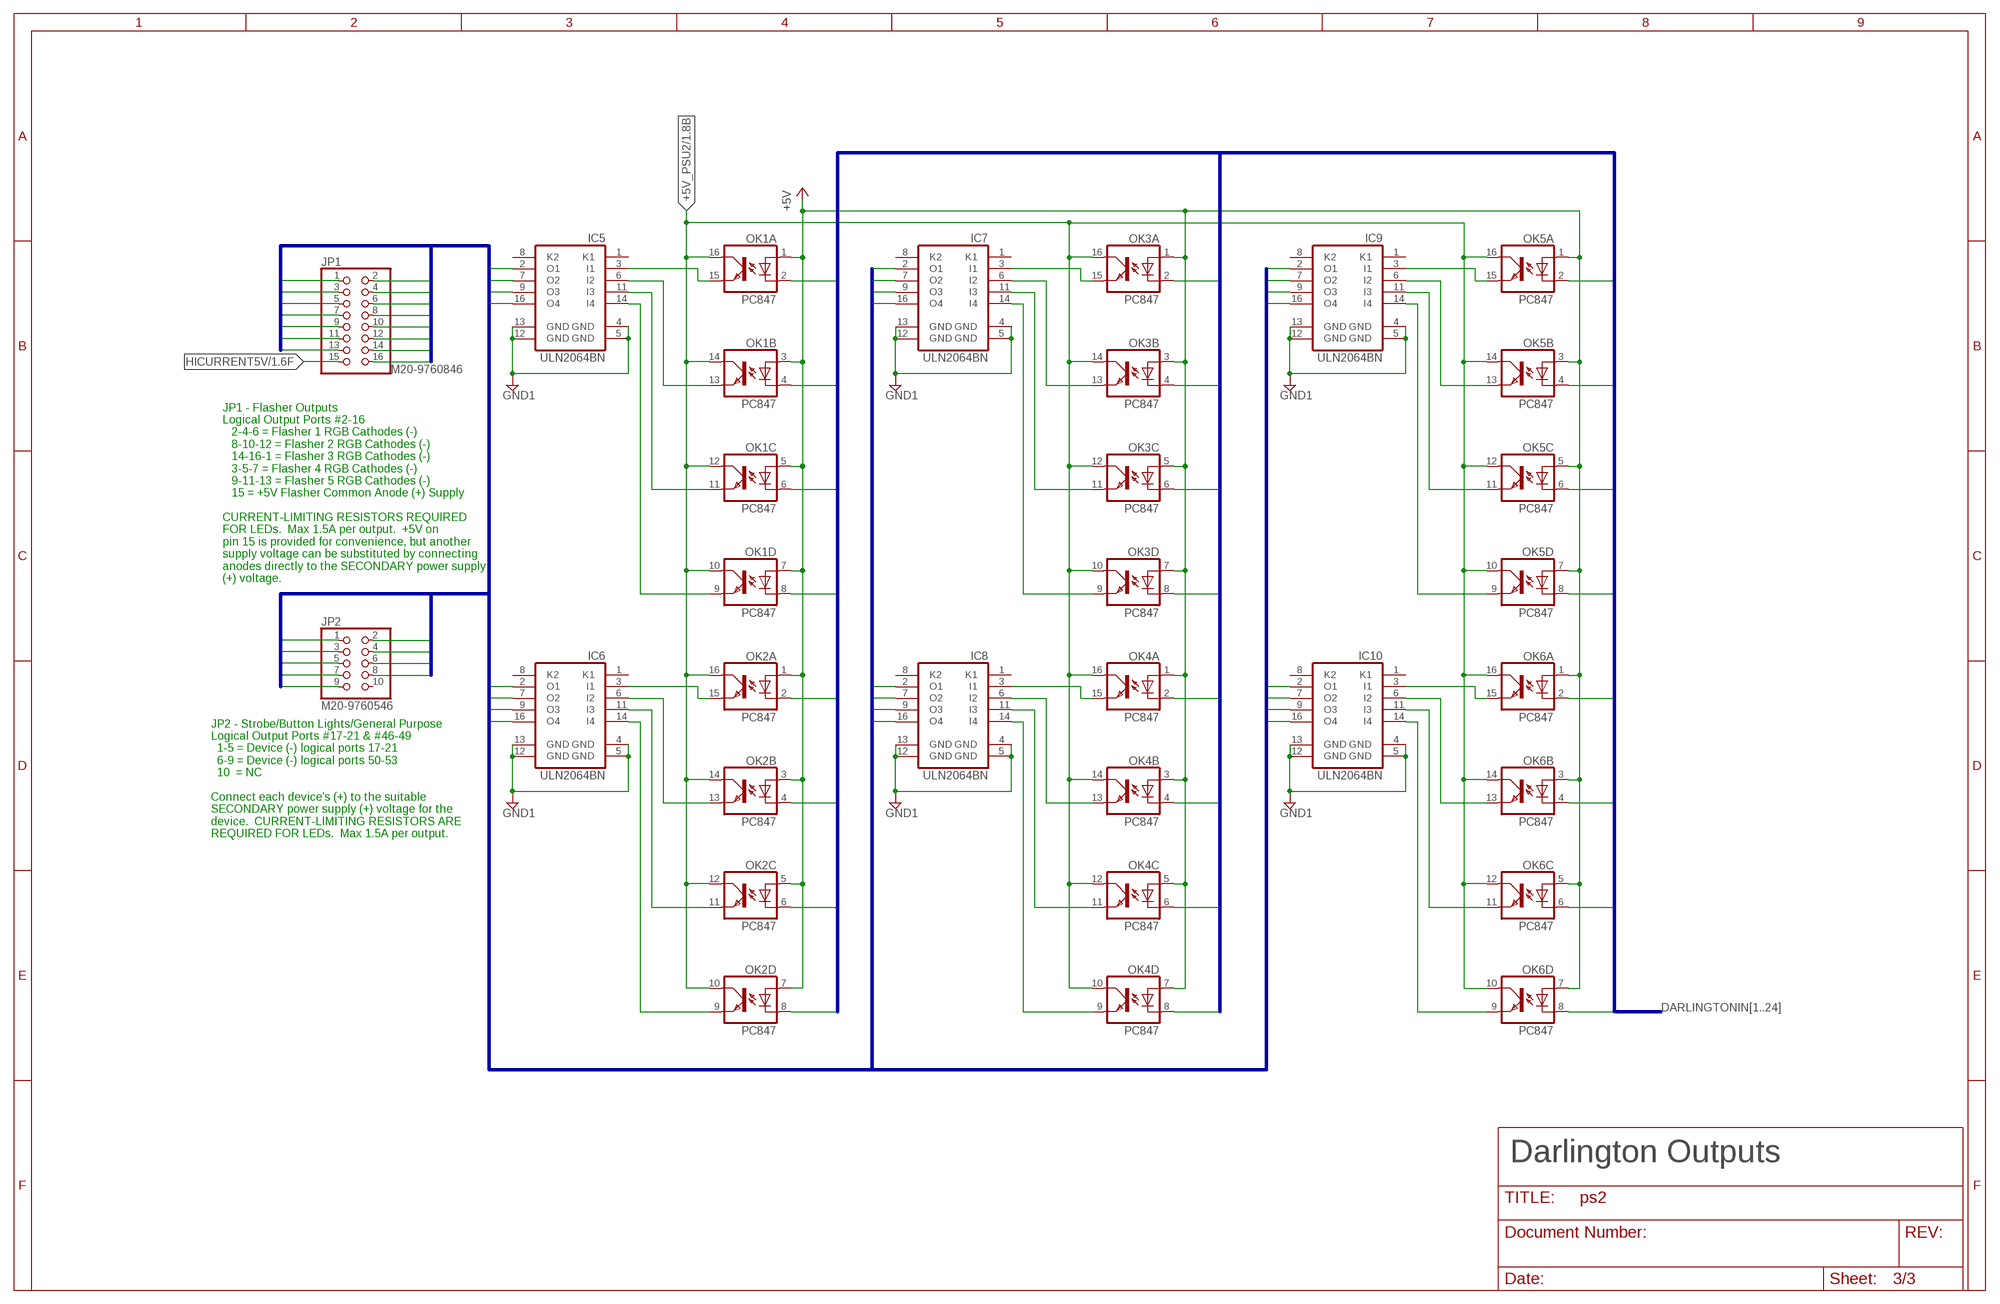
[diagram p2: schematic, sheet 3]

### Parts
IC5  ULN2064BN  [DIL16]
IC6  ULN2064BN  [DIL16]
IC7  ULN2064BN  [DIL16]
IC8  ULN2064BN  [DIL16]
IC9  ULN2064BN  [DIL16]
IC10  ULN2064BN  [DIL16]
JP1  M20-9760846  PINHD-2X8  [2X08]
JP2  M20-9760546  PINHD-2X5  [2X05]
OK1  PC847  [DIL16]
OK2  PC847  [DIL16]
OK3  PC847  [DIL16]
OK4  PC847  [DIL16]
OK5  PC847  [DIL16]
OK6  PC847  [DIL16]

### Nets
+5V [+5V]: OK1.1(A:A) OK1.3(B:A) OK1.5(C:A) OK1.7(D:A) OK2.1(A:A) OK2.3(B:A) OK2.5(C:A) OK2.7(D:A) OK3.1(A:A) OK3.3(B:A) OK3.5(C:A) OK3.7(D:A) OK4.1(A:A) OK4.3(B:A) OK4.5(C:A) OK4.7(D:A) OK5.1(A:A) OK5.3(B:A) OK5.5(C:A) OK5.7(D:A) OK6.1(A:A) OK6.3(B:A) OK6.5(C:A) OK6.7(D:A) ; also sheet 1,2
+5V_PSU2: OK1.10(D:COL) OK1.12(C:COL) OK1.14(B:COL) OK1.16(A:COL) OK2.10(D:COL) OK2.12(C:COL) OK2.14(B:COL) OK2.16(A:COL) OK3.10(D:COL) OK3.12(C:COL) OK3.14(B:COL) OK3.16(A:COL) OK4.10(D:COL) OK4.12(C:COL) OK4.14(B:COL) OK4.16(A:COL) OK5.10(D:COL) OK5.12(C:COL) OK5.14(B:COL) OK5.16(A:COL) OK6.10(D:COL) OK6.12(C:COL) OK6.14(B:COL) OK6.16(A:COL) ; also sheet 1
DARLINGTONIN1: OK1.2(A:C) ; also sheet 1
DARLINGTONIN2: OK1.4(B:C) ; also sheet 1
DARLINGTONIN3: OK1.6(C:C) ; also sheet 1
DARLINGTONIN4: OK1.8(D:C) ; also sheet 1
DARLINGTONIN5: OK2.2(A:C) ; also sheet 1
DARLINGTONIN6: OK2.4(B:C) ; also sheet 1
DARLINGTONIN7: OK2.6(C:C) ; also sheet 1
DARLINGTONIN8: OK2.8(D:C) ; also sheet 1
DARLINGTONIN9: OK3.2(A:C) ; also sheet 1
DARLINGTONIN10: OK3.4(B:C) ; also sheet 1
DARLINGTONIN11: OK3.6(C:C) ; also sheet 1
DARLINGTONIN12: OK3.8(D:C) ; also sheet 1
DARLINGTONIN13: OK4.2(A:C) ; also sheet 1
DARLINGTONIN14: OK4.4(B:C) ; also sheet 1
DARLINGTONIN15: OK4.6(C:C) ; also sheet 1
DARLINGTONIN16: OK4.8(D:C) ; also sheet 1
DARLINGTONIN17: OK5.2(A:C) ; also sheet 1
DARLINGTONIN18: OK5.4(B:C) ; also sheet 1
DARLINGTONIN19: OK5.6(C:C) ; also sheet 1
DARLINGTONIN20: OK5.8(D:C) ; also sheet 1
DARLINGTONIN21: OK6.2(A:C) ; also sheet 1
DARLINGTONIN22: OK6.4(B:C) ; also sheet 1
DARLINGTONIN23: OK6.6(C:C) ; also sheet 1
DARLINGTONIN24: OK6.8(D:C) ; also sheet 1
DARLINGTONOUT1 [Lamps]: IC5.2(O1) JP1.2
DARLINGTONOUT2 [Lamps]: IC5.7(O2) JP1.4
DARLINGTONOUT3 [Lamps]: IC5.9(O3) JP1.6
DARLINGTONOUT4 [Lamps]: IC5.16(O4) JP1.8
DARLINGTONOUT5 [Lamps]: IC6.2(O1) JP1.10
DARLINGTONOUT6 [Lamps]: IC6.7(O2) JP1.12
DARLINGTONOUT7 [Lamps]: IC6.9(O3) JP1.14
DARLINGTONOUT8 [Lamps]: IC6.16(O4) JP1.16
DARLINGTONOUT9 [Lamps]: IC7.2(O1) JP1.1
DARLINGTONOUT10 [Lamps]: IC7.7(O2) JP1.3
DARLINGTONOUT11 [Lamps]: IC7.9(O3) JP1.5
DARLINGTONOUT12 [Lamps]: IC7.16(O4) JP1.7
DARLINGTONOUT13 [Lamps]: IC8.2(O1) JP1.9
DARLINGTONOUT14 [Lamps]: IC8.7(O2) JP1.11
DARLINGTONOUT15 [Lamps]: IC8.9(O3) JP1.13
DARLINGTONOUT16 [Lamps]: IC8.16(O4) JP2.1
DARLINGTONOUT17 [Lamps]: IC9.2(O1) JP2.2
DARLINGTONOUT18 [Lamps]: IC9.7(O2) JP2.3
DARLINGTONOUT19 [Lamps]: IC9.9(O3) JP2.4
DARLINGTONOUT20 [Lamps]: IC9.16(O4) JP2.5
DARLINGTONOUT21 [Lamps]: IC10.2(O1) JP2.6
DARLINGTONOUT22 [Lamps]: IC10.7(O2) JP2.7
DARLINGTONOUT23 [Lamps]: IC10.9(O3) JP2.8
DARLINGTONOUT24 [Lamps]: IC10.16(O4) JP2.9
GND1 [Lamp Power & Ground]: IC5.4(GND) IC5.5(GND) IC5.12(GND) IC5.13(GND) IC6.4(GND) IC6.5(GND) IC6.12(GND) IC6.13(GND) IC7.4(GND) IC7.5(GND) IC7.12(GND) IC7.13(GND) IC8.4(GND) IC8.5(GND) IC8.12(GND) IC8.13(GND) IC9.4(GND) IC9.5(GND) IC9.12(GND) IC9.13(GND) IC10.4(GND) IC10.5(GND) IC10.12(GND) IC10.13(GND) ; also sheet 1
HICURRENT5V [Lamp Power & Ground]: JP1.15 ; also sheet 1
N$22: IC5.3(I1) OK1.15(A:EMIT)
N$23: IC5.6(I2) OK1.13(B:EMIT)
N$24: IC5.11(I3) OK1.11(C:EMIT)
N$25: IC5.14(I4) OK1.9(D:EMIT)
N$27: IC6.3(I1) OK2.15(A:EMIT)
N$28: IC6.6(I2) OK2.13(B:EMIT)
N$29: IC6.11(I3) OK2.11(C:EMIT)
N$30: IC6.14(I4) OK2.9(D:EMIT)
N$31: IC7.3(I1) OK3.15(A:EMIT)
N$32: IC7.6(I2) OK3.13(B:EMIT)
N$33: IC7.11(I3) OK3.11(C:EMIT)
N$35: IC7.14(I4) OK3.9(D:EMIT)
N$36: IC8.3(I1) OK4.15(A:EMIT)
N$37: IC8.6(I2) OK4.13(B:EMIT)
N$39: IC8.11(I3) OK4.11(C:EMIT)
N$40: IC8.14(I4) OK4.9(D:EMIT)
N$73: IC9.3(I1) OK5.15(A:EMIT)
N$77: IC9.6(I2) OK5.13(B:EMIT)
N$78: IC9.11(I3) OK5.11(C:EMIT)
N$79: IC9.14(I4) OK5.9(D:EMIT)
N$80: IC10.3(I1) OK6.15(A:EMIT)
N$81: IC10.6(I2) OK6.13(B:EMIT)
N$82: IC10.11(I3) OK6.11(C:EMIT)
N$83: IC10.14(I4) OK6.9(D:EMIT)
Unconnected: IC5.1(K1) IC5.8(K2) IC6.1(K1) IC6.8(K2) IC7.1(K1) IC7.8(K2) IC8.1(K1) IC8.8(K2) IC9.1(K1) IC9.8(K2) IC10.1(K1) IC10.8(K2) JP2.10

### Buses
DARLINGTONIN[1..24]
DARLINGTONOUT[1..24]

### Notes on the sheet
- JP1 - Flasher Outputs
  Logical Output Ports #2-16
     2-4-6 = Flasher 1 RGB Cathodes (-)
     8-10-12 = Flasher 2 RGB Cathodes (-)
     14-16-1 = Flasher 3 RGB Cathodes (-)
     3-5-7 = Flasher 4 RGB Cathodes (-)
     9-11-13 = Flasher 5 RGB Cathodes (-)
     15 = +5V Flasher Common Anode (+) Supply
  
  CURRENT-LIMITING RESISTORS REQUIRED
  FOR LEDs.  Max 1.5A per output.  +5V on
  pin 15 is provided for convenience, but another
  supply voltage can be substituted by connecting
  anodes directly to the SECONDARY power supply
  (+) voltage.
- JP2 - Strobe/Button Lights/General Purpose
  Logical Output Ports #17-21 & #46-49
    1-5 = Device (-) logical ports 17-21
    6-9 = Device (-) logical ports 50-53
    10  = NC
  
  Connect each device's (+) to the suitable 
  SECONDARY power supply (+) voltage for the 
  device.  CURRENT-LIMITING RESISTORS ARE
  REQUIRED FOR LEDs.  Max 1.5A per output.
- Darlington Outputs

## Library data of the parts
C1-C4 C6 C7 C9 C12 = rcl:C-US: CAPACITOR, American symbol
C5 C8 C10 C11 = rcl:CPOL-US: POLARIZED CAPACITOR, American symbol
D1 = diode:DIODE-: DIODE
FRDM1 = kl25z:FRDM-KL25Z: For creating FRDM-KL25Z shields
IC1-IC4 = tlc5940:TCL5940: 16-Channel 12-Bit LED Driver
IC5-IC10 = uln-udn:ULN2064B: DRIVER ARRAY
IC11 = maxim:ICM7555: TIMER; MF: MAXIM; MPN: ICM7555IPA+; OC_FARNELL: 9663762; OC_NEWARK: 68K4387
IC12 = v-reg:LD117A?*: Low drop fixed and adjustable positive voltage regulators 1 A Source: http://www.st.com/stonline/products/literature/ds/7194/ld1117axx.pdf
JP1 = pinhead:PINHD-2X8: PIN HEADER
JP2 = pinhead:PINHD-2X5: PIN HEADER
JP3 = pinhead:PINHD-2X9: PIN HEADER
JP4 = con-molex:KK-156-4: KK 156 HEADER Source: http://www.molex.com/pdm_docs/sd/026604100_sd.pdf; OC_FARNELL: unknown; OC_NEWARK: unknown
JP5 = pinhead:PINHD-2X13: PIN HEADER
JP6 JP9 = pinhead:PINHD-2X2: PIN HEADER
JP7 = pinhead:PINHD-2X4: PIN HEADER
JP8 = con-molex:22-23-2021: .100" (2.54mm) Center Header - 2 Pin; MF: MOLEX; MPN: 22-23-2021; OC_FARNELL: 1462926; OC_NEWARK: 25C3832
JP10 JP11 = pinhead:PINHD-2X6: PIN HEADER
JP12 = pinhead:PINHD-1X6: PIN HEADER
K1 = relay:G5V-2: OMRON PCB Relay Source: http://www.omron.com/ecb/products/pdf/en-g5v2.pdf; MPN: G5V-2 5DC; OC_FARNELL: 9949488; OC_NEWARK: 78K5703
OK1-OK12 = optocoupler:PC847: SHARP OPTO COUPLER; OC_FARNELL: 9707735; OC_NEWARK: unknown
OK13-OK15 = optocoupler:PC817: SHARP OPTO COUPLER; MPN: PC817X4J000F; OC_FARNELL: 9707727; OC_NEWARK: 97K7059
Q7A Q7B Q7C Q7D Q8A Q8B Q8C Q8D Q9A Q9B Q9C Q9D Q10A Q10B Q10C Q10D Q11A Q11B Q11C Q11D Q12A Q12B Q12C Q12D = BUK7575:BUK7575-55A
R1-R44 R46 R47 R49 = resistor:R-US_: RESISTOR, American symbol
R45 R48 = rcl:R-US_: RESISTOR, American symbol
T1 T3 T4 T6 = transistor-neu-to92:*-NPN-: NPN Transistror
T2 T5 = transistor-neu-to92:*-PNP-: PNP Transistror
U$1-U$4 = NetJumper:NETJUMPER

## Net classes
1 MOSFET Power & Ground: width 1.575 mm
2 Lamps: width 0.305 mm
3 Lamp Power & Ground: width 2.032 mm
4 +5V: width 0.457 mm
5 GND: width 0.457 mm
